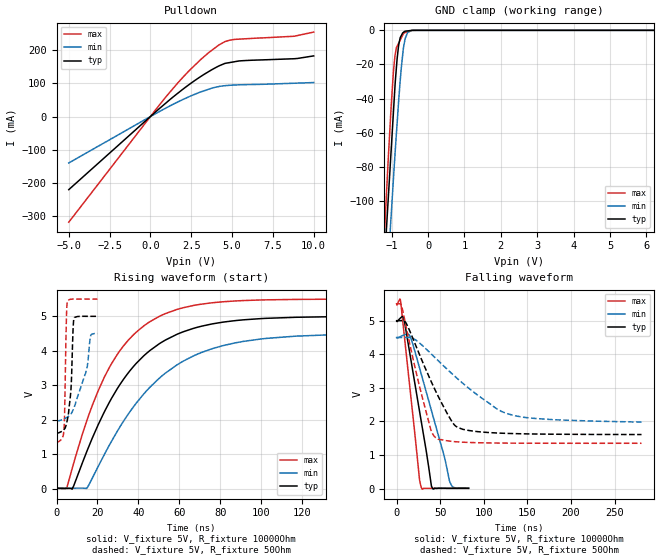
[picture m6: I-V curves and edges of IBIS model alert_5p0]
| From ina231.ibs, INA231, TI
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|   alert_5p0 Model
[Model]   alert_5p0
Model_type   Open_drain
Polarity   Non-Inverting
Vmeas = 2.5
Vref = 5.0
Cref = 2pF
Rref = 10000
|   typ   min   max
|   (nom PVT)   (fast PVT)   (slow PVT)
|C_comp from frequency sweep method (F=50KHz)
|C_comp   2.417e-10   1.981e-10   4.401e-10
|ON state : BUFFER OUTPUT TURNED LOW
|C_comp   2.417e-10   1.981e-10   4.401e-10
|OFF state: BUFFER IN HIGH IMPEDANCE
|C_comp   2.247e-12   1.898e-12   2.626e-12
|C_comp from LC tank measurement(L=1nH)
|Resonant Frequency(Hz)   5.880e+09   5.890e+09   5.670e+09
C_comp   7.334e-13   7.309e-13   7.887e-13
|ON state : BUFFER OUTPUT TURNED LOW
|Resonant Frequency(Hz)   5.880e+09   5.890e+09   5.670e+09
|C_comp   7.334e-13   7.309e-13   7.887e-13
|OFF state: BUFFER IN HIGH IMPEDANCE
|Resonant Frequency(Hz)   5.100e+09   5.820e+09   4.670e+09
|C_comp   9.748e-13   7.486e-13   1.163e-12
| Where nom  PVT is Nominal Process, 5V, 27C
|   Fast PVT is Strong Process,  5.5V, -40C
|   Slow PVT is Weak Process,   4.5V, 125C
[Voltage Range]   5   4.5   5.5
|Ambient Temperature   25   150   -65
|Junction Temperature
[Temperature Range]   27   125   -40
[Pullup Reference]   5   4.5   5.5
[Pulldown Reference]   0   0   0
[Power Clamp Reference]   5   4.5   5.5
[GND Clamp Reference]   0   0   0
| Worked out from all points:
|   slope of the pulldown table from 0 to 0.75 V, typ, clamps not added: 23.2 ohm
|   GND clamp passes 1 mA (typ) near -0.67 V on its own axis
|   falling waveform, V_fixture 5V, R_fixture 10000Ohm: 20-80 % time 19.3ns typ, 28.9ns min, 13.6ns max; typ from 5 V to 0.012 V
|   rising waveform, V_fixture 5V, R_fixture 10000Ohm: 20-80 % time 31.2ns typ, 36.5ns min, 26.4ns max; typ from 0.011 V to 5 V
|   falling waveform, V_fixture 5V, R_fixture 50Ohm: 20-80 % time 36ns typ, 68.8ns min, 22.8ns max; typ from 5 V to 1.61 V
|   rising waveform, V_fixture 5V, R_fixture 50Ohm: 20-80 % time 1.86ns typ, 6.55ns min, 780ps max; typ from 1.61 V to 5 V
[Pulldown]
|   Voltage   I(typ)   I(min)   I(max)
-5V       -220.2mA   -139.8mA   -318.3mA
968mV     41.53mA    26.15mA    60.34mA
2.376V    96.53mA    59.97mA    138.2mA
3.547V    134.8mA    81.88mA    191.6mA
4.186V    152.2mA    90.35mA    215.3mA
4.565V    160.1mA    92.99mA    225.7mA
4.851V    162.6mA    94.18mA    230mA
5.66V     168.3mA    95.89mA    233.8mA
8.806V    174.2mA    100.4mA    241.9mA
10V       182.7mA    102.4mA    254.4mA
[GND Clamp]
|   Voltage   I(typ)   I(min)   I(max)
-5V       -1.676A    -1.624A    -1.761A
-1.216V   -145.1mA   -181.2mA   -126.8mA
-1.14V    -115.4mA   -153.7mA   -95.04mA
-1.026V   -74.77mA   -112.9mA   -49.45mA
-951.5mV  -48.22mA   -87.39mA   -24.53mA
-907.5mV  -32.54mA   -72.67mA   -14.72mA
-805mV    -8.37mA    -40.67mA   -7.412mA
-684mV    -1.305mA   -11.71mA   -2.26mA
-630mV    -510uA     -4.897mA   -1.325mA
-558mV    -323.4uA   -1.22mA    -810uA
-351mV    -3.632uA   -6.319uA   -4.803uA
10V       0A         0A         0A
[POWER Clamp]
|   Voltage   I(typ)   I(min)   I(max)
-5V       0A         0A         0A
0V        0A         0A         0A
10V       0A         0A         0A
[Ramp]
R_load = 10000
|   typ   min   max
dV/dt_r   2.99325/3.11731e-08   2.69036/3.65017e-08   3.29489/2.63643e-08
dV/dt_f   2.99324/1.93552e-08   2.69026/2.89375e-08   3.29489/1.35623e-08
[Falling Waveform]
V_fixture = 5V
V_fixture_min = 4.5V
V_fixture_max = 5.5V
R_fixture = 10000Ohm
|   Time   V(typ)   V(min)   V(max)
0s        5V         4.5V       5.5V
4.55ns    5.084V     4.531V     5.587V
8.1ns     5.08V      4.572V     4.733V
15.45ns   3.982V     4.534V     2.951V
26.25ns   2.312V     3.6V       276.6mV
28.6ns    1.95V      3.381V     17.12mV
39.9ns    82.88mV    2.33V      10.13mV
40.85ns   23.23mV    2.242V     10.03mV
62.6ns    13.35mV    113.8mV    9.114mV
82.6ns    11.62mV    18.27mV    8.605mV
[Rising Waveform]
V_fixture = 5V
V_fixture_min = 4.5V
V_fixture_max = 5.5V
R_fixture = 10000Ohm
|   Time   V(typ)   V(min)   V(max)
0s        11.24mV    16.04mV    8.512mV
5.05ns    6.284mV    12.78mV    29.15mV
7.65ns    -15.74mV   13.29mV    583.9mV
14.7ns    1.063V     3.62mV     1.955V
23.25ns   2.214V     978.4mV    3.22V
30.35ns   2.963V     1.73V      3.952V
50.15ns   4.202V     3.201V     4.998V
68.3ns    4.674V     3.889V     5.33V
91.4ns    4.899V     4.273V     5.458V
189.5ns   5V         4.5V       5.5V
[Falling Waveform]
V_fixture = 5V
V_fixture_min = 4.5V
V_fixture_max = 5.5V
R_fixture = 50Ohm
|   Time   V(typ)   V(min)   V(max)
0s        5V         4.5V       5.5V
5.05ns    5.003V     4.501V     5.488V
11.05ns   4.922V     4.501V     4.802V
25.15ns   4.061V     4.361V     3.165V
39.3ns    3.209V     4.022V     1.75V
47.45ns   2.763V     3.817V     1.477V
62.3ns    2.046V     3.451V     1.411V
70.35ns   1.821V     3.263V     1.393V
126.8ns   1.646V     2.233V     1.357V
280.9ns   1.612V     1.982V     1.352V
[Rising Waveform]
V_fixture = 5V
V_fixture_min = 4.5V
V_fixture_max = 5.5V
R_fixture = 50Ohm
|   Time   V(typ)   V(min)   V(max)
0s        1.612V     1.964V     1.353V
3.65ns    1.716V     2.023V     1.717V
4ns       1.739V     2.033V     2.323V
4.85ns    1.882V     2.059V     4.984V
5.3ns     2.001V     2.076V     5.435V
7.05ns    2.875V     2.164V     5.497V
8.45ns    4.916V     2.336V     5.501V
14.85ns   5V         3.496V     5.5V
16.8ns    5V         4.461V     5.5V
20ns      5V         4.5V       5.5V
